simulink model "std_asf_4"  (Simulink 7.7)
settings: Solver=ode45  StartTime=0.0  StopTime=10.0  RelTol=1e-3

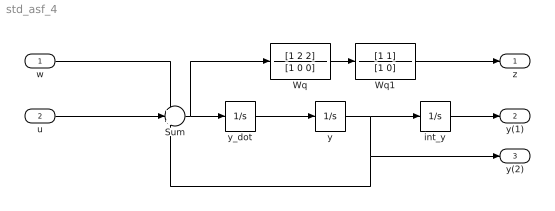
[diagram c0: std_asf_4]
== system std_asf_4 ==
  w : Inport
  u : Inport  Port=2
  Sum : Sum  Inputs=+++
  Wq : TransferFcn  Numerator=[1 2 2]  Denominator=[1 0 0]
  Wq1 : TransferFcn  Numerator=[1 1]  Denominator=[1 0]
  int_y : Integrator
  y : Integrator
  y_dot : Integrator  InitialCondition=-1
  z : Outport
  y(1) : Outport  Port=2
  y(2) : Outport  Port=3
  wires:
  Sum/1 -> y_dot/1, Wq/1
  y_dot/1 -> y/1
  y/1 -> Sum/3, y(2)/1, int_y/1
  Wq/1 -> Wq1/1
  w/1 -> Sum/1
  u/1 -> Sum/2
  Wq1/1 -> z/1
  int_y/1 -> y(1)/1
